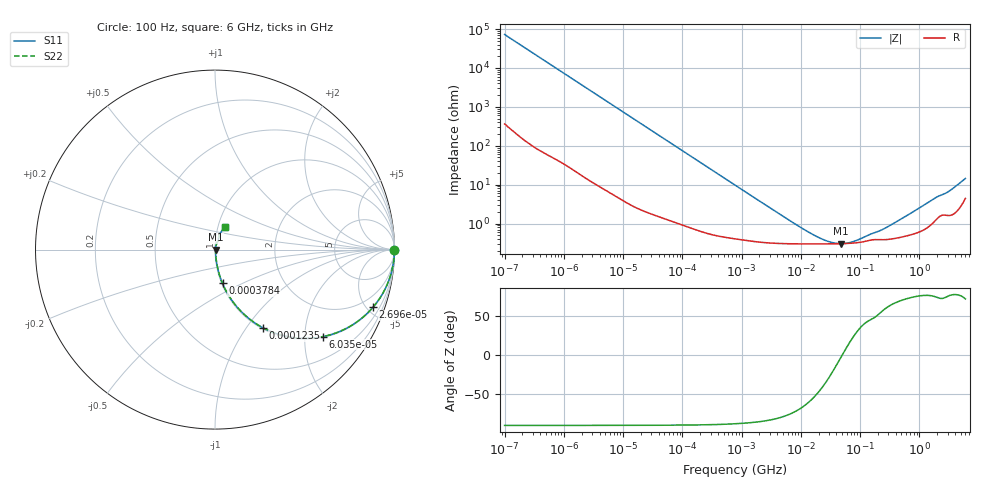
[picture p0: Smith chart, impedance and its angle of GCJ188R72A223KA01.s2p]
!Murata Part Number: GCJ188R72A223KA01
!These Parameters are Measured in Series Mode Connection
!Data Generated on Mar 13, 2026
!  o--ll--o
!Port1  Port2
!  o------o
!Operation Temp=25[degC], DC Bias Voltage=0[V]
!Freq. Start=100[Hz] Stop=6[GHz] 401[Steps]
# Hz S RI R 50
!Freq.(Hz) S11(Real) S11(Imag) S21(Real) S21(Imag) S12(Real) S12(Imag) S22(Real) S22(Imag)
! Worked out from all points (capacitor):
!   401 points, 100 Hz to 6 GHz, reference 50 ohm
!   read as one part in series: C = 21.9 nF near 109 Hz
!   lowest |Z| = 303 mohm at 47.65 MHz (marker M1)
!   series resonance near 49.7 MHz, so ESL is about 470 pH
!   S11 on the Smith chart (normalised r, x): 100 Hz: open; 26.96 kHz: 1.04, -5.47; 60.35 kHz: 1.02, -2.45; 123.5 kHz: 1.02, -1.20; 378.4 kHz: 1.01, -0.39; 6 GHz: 1.09, +0.27
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100  1 -0.00138  8.8e-06 0.00138  8.8e-06 0.00138  1 -0.00138
2008  0.9991 -0.0274  0.00088 0.0274  0.00088 0.0274  0.9991 -0.0274
8801  0.9853 -0.1179  0.0147 0.1179  0.0147 0.1179  0.9853 -0.1179
16473  0.9512 -0.2126  0.0488 0.2126  0.0488 0.2126  0.9512 -0.2126
26957  0.8803 -0.3212  0.1197 0.3212  0.1197 0.3212  0.8803 -0.3212
40335  0.7682 -0.418  0.2318 0.418  0.2318 0.418  0.7682 -0.418
60352  0.5992 -0.4852  0.4008 0.4852  0.4008 0.4852  0.5992 -0.4852
86348  0.4248 -0.4886  0.5752 0.4886  0.5752 0.4886  0.4248 -0.4886
123542  0.268 -0.4362  0.732 0.4362  0.732 0.4362  0.268 -0.4362
202169  0.1236 -0.3207  0.8764 0.3207  0.8764 0.3207  0.1236 -0.3207
378399  0.0418 -0.1882  0.9582 0.1882  0.9582 0.1882  0.0418 -0.1882
774597  0.0132 -0.0952  0.9868 0.0952  0.9868 0.0952  0.0132 -0.0952
2481164  0.00413 -0.0303  0.9959 0.0303  0.9959 0.0303  0.00413 -0.0303
1.555665e7  0.003 -0.00439  0.997 0.00439  0.997 0.00439  0.003 -0.00439
2.911731e7  0.00299 -0.00171  0.997 0.00171  0.997 0.00171  0.00299 -0.00171
4.764863e7  0.00302 -0.000128  0.997 0.000128  0.997 0.000128  0.00302 -0.000128
6.233367e7  0.00307 0.000695  0.9969 -0.000695  0.9969 -0.000695  0.00307 0.000695
8.527865e7  0.00318 0.00172  0.9968 -0.00172  0.9968 -0.00172  0.00318 0.00172
3.124326e8  0.00397 0.00774  0.996 -0.00774  0.996 -0.00774  0.00397 0.00774
1.791126e9  0.0128 0.0417  0.9872 -0.0417  0.9872 -0.0417  0.0128 0.0417
3.065283e9  0.0196 0.0611  0.9804 -0.0611  0.9804 -0.0611  0.0196 0.0611
6e9  0.0585 0.1236  0.9415 -0.1236  0.9415 -0.1236  0.0585 0.1236
